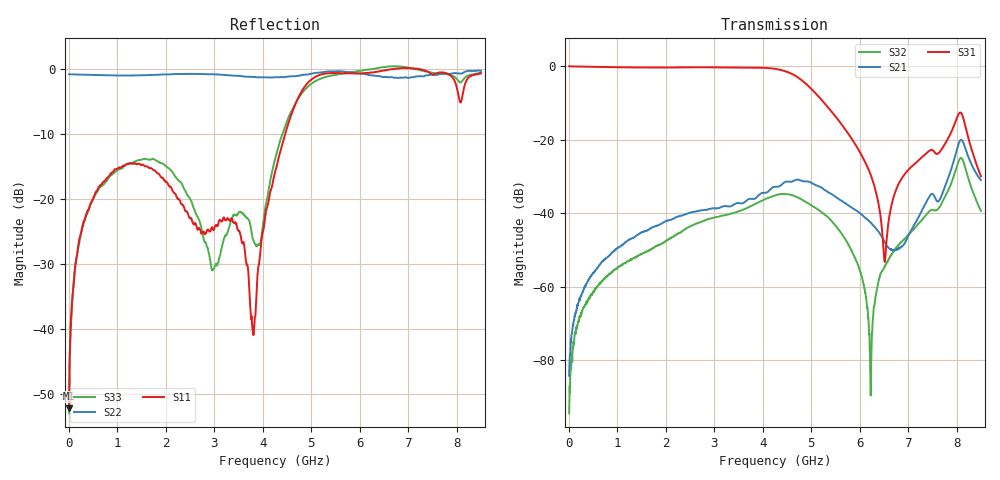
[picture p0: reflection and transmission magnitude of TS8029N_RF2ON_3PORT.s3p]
!Created with skrf (http://scikit-rf.org).
# GHz S RI R 50.0
!freq ReS11 ImS11 ReS12 ImS12 ReS13 ImS13
! ReS21 ImS21 ReS22 ImS22 ReS23 ImS23
! ReS31 ImS31 ReS32 ImS32 ReS33 ImS33
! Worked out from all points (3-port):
!   1601 points, 10 MHz to 8.5 GHz, reference 50 ohm
!   strongest paths, dB at 10 MHz, 2.132 GHz, 4.255 GHz, 6.378 GHz, 8.5 GHz:
!     S31: -0.1, -0.4, -0.8, -36.7, -30.0
!     S21: -84.3, -41.7, -32.9, -44.9, -31.0
!     S32: -94.5, -46.6, -35.2, -59.4, -39.4
!   lowest |S11| = -52.1 dB at 10 MHz (marker M1), VSWR 1.00, Z = 50.1 + j0.232 ohm
!   |S11| at or under -10 dB: start of sweep to 4.463 GHz
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0.01  0.000873 0.00231  4.9e-05 4.26e-05  0.994 -0.011
      4.28e-05 4.38e-05  -0.918 0.00381  1.57e-05 2.1e-05
      0.9939 -0.0109  3.47e-06 1.86e-05  0.00221 0.000496
0.2487813  0.00245 -0.0541  7.62e-05 0.000745  0.968 -0.1553
           8.67e-05 0.000741  -0.9088 0.0642  -3.83e-05 -0.00041
           0.9684 -0.1552  -4.41e-05 -0.000387  -0.00236 -0.0525
0.9067563  -0.0802 -0.1407  -2.88e-05 0.00294  0.8137 -0.5164
           -5.14e-05 0.00295  -0.8672 0.2402  -0.00136 -0.000891
           0.8137 -0.5163  -0.00133 -0.000851  -0.0688 -0.14
3.803969  0.00554 -0.00785  0.01 0.0118  -0.8551 -0.417
          0.0101 0.0119  -0.4721 0.7379  0.000498 0.0129
          -0.855 -0.4176  0.000498 0.0129  -0.0051 -0.0489
4.255  -0.1245 0.1023  0.0192 0.0123  -0.911 0.0853
       0.0192 0.0123  -0.3302 0.8049  0.0107 0.0137
       -0.9105 0.0853  0.0106 0.0138  0.1986 0.0436
5.677075  0.8909 -0.2754  0.00987 -0.00985  0.0725 0.1259
          0.00984 -0.00986  -0.049 0.96  0.00264 -0.00388
          0.0725 0.1259  0.00261 -0.00389  0.6292 -0.6858
6.228925  0.779 -0.5357  0.00508 -0.00539  0.0234 0.0232
          0.00512 -0.00538  0.0216 0.9011  5.42e-05 2.86e-05
          0.0234 0.0232  3.26e-05 5.31e-06  0.3516 -0.9361
6.515462  0.7233 -0.665  0.00325 -0.00243  -0.00113 0.00181
          0.00325 -0.00239  0.1285 0.8646  -2.3e-05 0.00188
          -0.00118 0.00182  -6.01e-06 0.00188  0.3403 -0.9866
8.059581  0.2691 -0.51  0.0935 0.00531  -0.1339 0.1878
          0.0938 0.00537  0.5156 0.7725  0.0539 -0.00383
          -0.1339 0.1878  0.0537 -0.00376  0.1574 -0.7845
8.5  0.6116 -0.7011  0.00459 -0.0277  0.0272 0.0161
     0.00453 -0.0277  0.5635 0.7952  -0.00149 -0.0106
     0.0273 0.0162  -0.00145 -0.0106  0.0418 -0.9463
